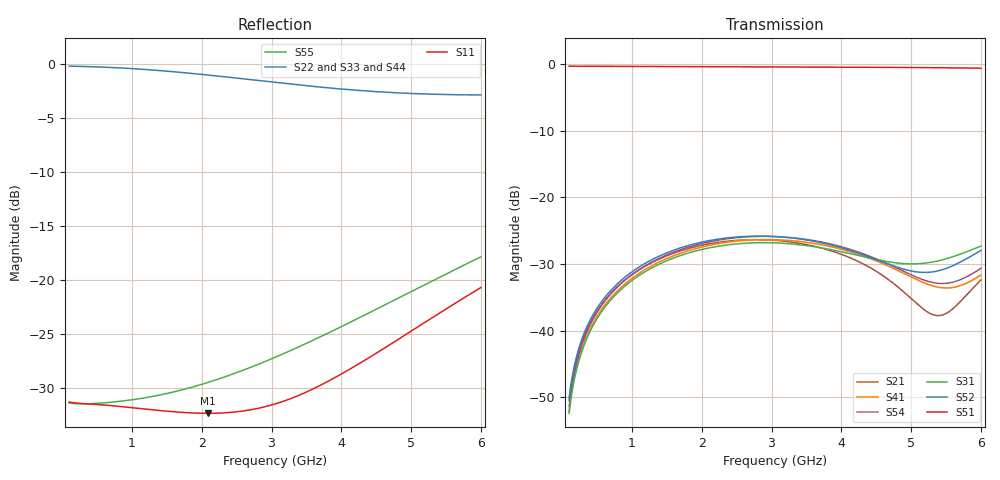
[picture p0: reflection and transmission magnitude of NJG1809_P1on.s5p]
! Port1:P1  Port2:P2  Port3:P3  Port4:P4  Port5:PC
# hz S ma R 50
! 5 Port Network Data from SP1.SP block
! freq  magS11  angS11  magS12  angS12  magS13  angS13  magS14  angS14
!  magS15  angS15
!  magS21  angS21  magS22  angS22  magS23  angS23
!  magS24  angS24  magS25  angS25
!  magS31  angS31  magS32  angS32
!  magS33  angS33  magS34  angS34  magS35  angS35
!  magS41  angS41
!  magS42  angS42  magS43  angS43  magS44  angS44  magS45  angS45
!  magS51  angS51  magS52  angS52  magS53  angS53  magS54  angS54
!  magS55  angS55
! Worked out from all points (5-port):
!   591 points, 100 MHz to 6 GHz, reference 50 ohm
!   strongest paths, dB at 100 MHz, 1.57 GHz, 3.05 GHz, 4.53 GHz, 6 GHz:
!     S51: -0.4, -0.4, -0.5, -0.5, -0.7
!     S52: -50.1, -28.0, -25.9, -29.4, -28.0
!     S31: -52.4, -29.2, -26.8, -29.4, -27.3
!     S54: -51.3, -28.3, -25.9, -29.4, -30.7
!     S41: -52.0, -28.9, -26.4, -29.7, -31.7
!     S21: -50.5, -28.5, -26.5, -31.3, -32.4
!   lowest |S11| = -32.3 dB at 2.09 GHz (marker M1), VSWR 1.05, Z = 51.1 - j2.18 ohm
!   |S11| at or under -10 dB: start of sweep to end of sweep
